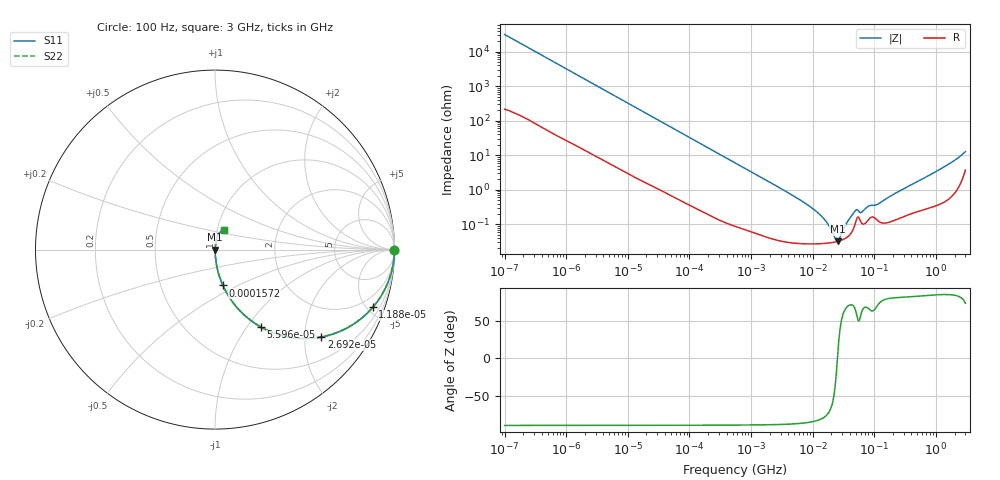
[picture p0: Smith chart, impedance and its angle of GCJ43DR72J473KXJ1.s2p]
!Murata Part Number: GCJ43DR72J473KXJ1
!These Parameters are Measured in Series Mode Connection
!Data Generated on Mar 13, 2026
!  o--ll--o
!Port1  Port2
!  o------o
!Operation Temp=25[degC], DC Bias Voltage=0[V]
!Freq. Start=100[Hz] Stop=3[GHz] 401[Steps]
# Hz S RI R 50
!Freq.(Hz) S11(Real) S11(Imag) S21(Real) S21(Imag) S12(Real) S12(Imag) S22(Real) S22(Imag)
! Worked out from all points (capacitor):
!   401 points, 100 Hz to 3 GHz, reference 50 ohm
!   read as one part in series: C = 50.4 nF near 109 Hz
!   lowest |Z| = 32 mohm at 25.25 MHz (marker M1)
!   series resonance near 25.17 MHz, so ESL is about 790 pH
!   S11 on the Smith chart (normalised r, x): 100 Hz: open; 11.88 kHz: 1.05, -5.45; 26.92 kHz: 1.02, -2.42; 55.95 kHz: 1.01, -1.17; 157.2 kHz: 1.00, -0.42; 3 GHz: 1.07, +0.24
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100  1 -0.00317  3.18e-05 0.00317  3.18e-05 0.00317  1 -0.00317
1788  0.9964 -0.0556  0.00358 0.0556  0.00358 0.0556  0.9964 -0.0556
4812  0.9769 -0.1457  0.0231 0.1457  0.0231 0.1457  0.9769 -0.1457
11882  0.8791 -0.3215  0.1209 0.3215  0.1209 0.3215  0.8791 -0.3215
26919  0.5928 -0.4864  0.4072 0.4864  0.4072 0.4864  0.5928 -0.4864
31977  0.5092 -0.4949  0.4908 0.4949  0.4908 0.4949  0.5092 -0.4949
55955  0.2567 -0.4317  0.7433 0.4317  0.7433 0.4317  0.2567 -0.4317
157206  0.0441 -0.1997  0.9559 0.1997  0.9559 0.1997  0.0441 -0.1997
547723  0.00452 -0.0602  0.9955 0.0602  0.9955 0.0602  0.00452 -0.0602
9794414  0.000279 -0.00293  0.9997 0.00293  0.9997 0.00293  0.000279 -0.00293
1.572531e7  0.000282 -0.00132  0.9997 0.00132  0.9997 0.00132  0.000282 -0.00132
2.316512e7  0.000308 -0.000228  0.9997 0.000228  0.9997 0.000228  0.000308 -0.000228
2.52476e7  0.00032 8.5e-06  0.9997 -8.5e-06  0.9997 -8.5e-06  0.00032 8.5e-06
2.751729e7  0.000334 0.000248  0.9997 -0.000248  0.9997 -0.000248  0.000334 0.000248
3.562563e7  0.000417 0.00102  0.9996 -0.00102  0.9996 -0.00102  0.000417 0.00102
4.815176e7  0.00096 0.00218  0.999 -0.00218  0.999 -0.00218  0.00096 0.00218
6.234031e7  0.00107 0.00197  0.9989 -0.00197  0.9989 -0.00197  0.00107 0.00197
8.070971e7  0.00138 0.00306  0.9986 -0.00306  0.9986 -0.00306  0.00138 0.00306
1.138854e8  0.00128 0.00361  0.9987 -0.00361  0.9987 -0.00361  0.00128 0.00361
1.751444e8  0.00119 0.00617  0.9988 -0.00617  0.9988 -0.00617  0.00119 0.00617
1.268426e9  0.00591 0.0424  0.9941 -0.0424  0.9941 -0.0424  0.00591 0.0424
3e9  0.0492 0.1118  0.9508 -0.1118  0.9508 -0.1118  0.0492 0.1118
